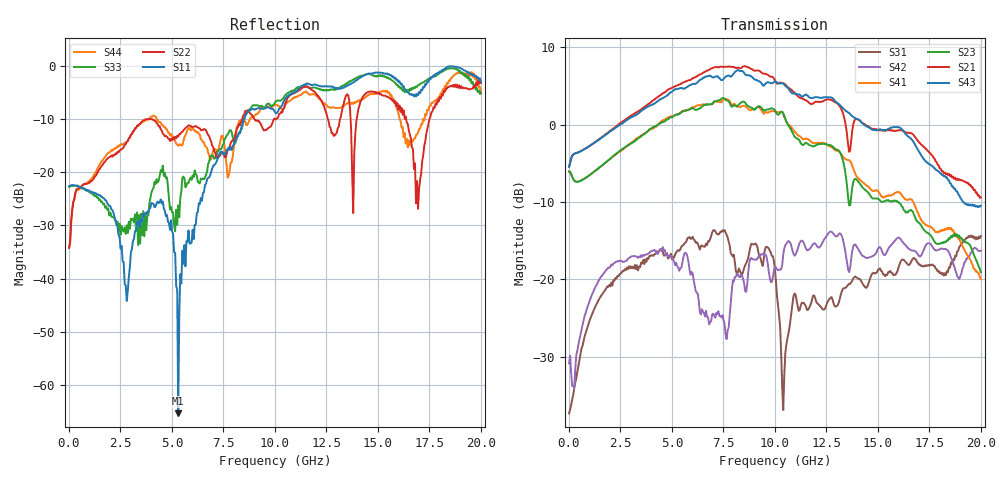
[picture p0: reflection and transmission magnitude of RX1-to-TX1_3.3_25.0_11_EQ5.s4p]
!Agilent Technologies,N5225A,MY51451112,A.09.50.13
!Agilent N5225A: A.09.50.13
!Date: Wednesday, January 31, 2018 11:03:44
!Correction: S11(Full 4 Port(1,2,3,4))
!S12(Full 4 Port(1,2,3,4))
!S13(Full 4 Port(1,2,3,4))
!S14(Full 4 Port(1,2,3,4))
!S21(Full 4 Port(1,2,3,4))
!S22(Full 4 Port(1,2,3,4))
!S23(Full 4 Port(1,2,3,4))
!S24(Full 4 Port(1,2,3,4))
!S31(Full 4 Port(1,2,3,4))
!S32(Full 4 Port(1,2,3,4))
!S33(Full 4 Port(1,2,3,4))
!S34(Full 4 Port(1,2,3,4))
!S41(Full 4 Port(1,2,3,4))
!S42(Full 4 Port(1,2,3,4))
!S43(Full 4 Port(1,2,3,4))
!S44(Full 4 Port(1,2,3,4))
!S4P File: Measurements: <S11,S12,S13,S14>,
!<S21,S22,S23,S24>,
!<S31,S32,S33,S34>,
!<S41,S42,S43,S44>:
# Hz S  RI  R 50
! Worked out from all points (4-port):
!   401 points, 10 MHz to 20 GHz, reference 50 ohm
!   strongest paths, dB at 10 MHz, 5.008 GHz, 10.01 GHz, 15 GHz, 20 GHz:
!     S43: -5.5, 4.3, 5.6, -0.7, -10.5
!     S21: -5.4, 4.8, 5.7, -0.6, -9.4
!     S23: -6.1, 1.0, 1.9, -9.5, -19.1
!     S41: -6.1, 1.1, 1.7, -8.5, -19.9
!     S42: -30.8, -17.3, -18.4, -16.0, -16.3
!     S31: -37.3, -17.4, -18.8, -18.8, -14.4
!   lowest |S11| = -65.4 dB at 5.307 GHz (marker M1), VSWR 1.00, Z = 49.9 + j0.0184 ohm
!   |S11| at or under -10 dB: start of sweep to 8.49 GHz
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1e7  -0.0743 -0.00292  -8.89e-05 0.000468  0.0139 0.000742  2.92e-05 0.000404
     0.5367 0.009  -0.0135 0.0141  -0.4973 0.00227  0.0265 0.0123
     0.0136 0.000496  -0.00028 0.000706  -0.0732 -0.00413  -0.000127 0.000166
     -0.4977 0.00338  0.0262 0.0118  0.5336 0.00844  -0.0131 0.0143
5.30735e9  -0.000503 0.000184  0.0287 -0.00434  0.0934 0.1368  0.0296 -0.014
           -0.7624 -1.635  0.1247 -0.1786  0.6923 0.935  0.1222 0.0089
           0.0883 0.1268  0.0331 -0.00106  0.0411 0.0266  0.0407 -0.0104
           0.9383 0.7056  0.119 0.0143  -1.269 -1.133  0.0639 -0.1666
7.156425e9  -0.0175 0.1237  0.0161 -0.0198  0.1315 0.0829  0.00209 -0.0334
            -2.353 0.1591  0.1221 -0.0682  1.377 -0.3481  0.0496 0.0277
            0.1668 0.1095  0.0249 -0.0277  0.0174 0.1358  0.00974 -0.0489
            1.104 -0.8915  0.0603 -0.00738  -1.732 1.089  0.1099 -0.1209
8.8056e9  0.0149 0.3867  0.0119 -0.0145  0.1162 0.094  -0.00669 -0.0154
          -0.6559 2.209  -0.0901 0.3462  0.1768 -1.281  0.0305 0.1286
          0.1283 0.0978  0.00122 -0.0238  0.0603 0.3911  -0.0145 -0.0259
          -0.397 -1.172  -0.0015 0.1368  0.5455 1.992  0.2561 0.2
1.270365e10  0.2708 0.5923  -0.0373 -0.00976  0.0236 0.0657  -0.031 0.00773
             1.276 -0.6872  0.1615 0.2084  -0.5745 0.4601  0.1837 0.1039
             0.0252 0.072  -0.0307 -0.0104  0.3927 0.4545  -0.0426 -0.00187
             -0.1644 0.7011  0.1777 0.1005  0.395 -1.449  0.2446 -0.3302
1.665168e10  0.5192 0.1367  -0.0277 0.0163  -0.0552 0.1094  -0.00317 0.0373
             -0.7956 -0.368  0.00913 0.1727  0.2263 0.16  0.094 0.1115
             -0.0592 0.1197  -0.0261 0.00433  0.6021 -0.1766  -0.00835 0.037
             0.3033 -0.1213  0.1074 0.1098  -0.5273 0.6017  -0.1115 -0.1625
2e10  0.7124 0.0631  0.0231 0.0348  -0.0787 0.1659  0.0345 0.0209
      -0.0431 0.3359  0.6933 0.0759  0.0684 -0.0881  0.1524 0.0426
      -0.0807 0.1726  0.00632 0.0478  0.5659 -0.0296  0.0476 0.0206
      -0.0593 -0.0813  0.1461 0.046  0.2622 0.1449  -0.1528 -0.5329
